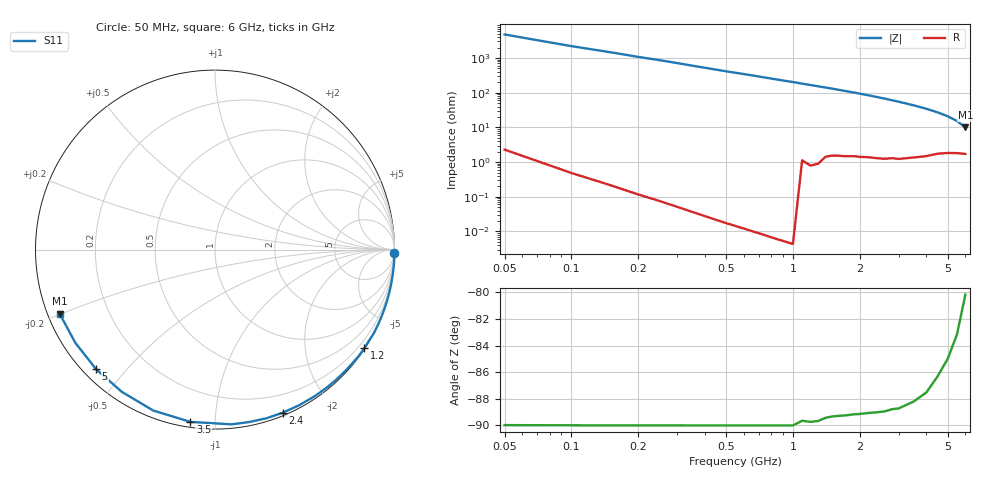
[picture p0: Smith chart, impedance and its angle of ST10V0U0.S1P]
! SIEMENS Discrete & RF Semiconductors
! BA892
! Si PIN Diode in SCD-80
! VR = 10 V
! S-Parameters:  September  1997
# GHz  S  MA  R  50
!  f  S11
! GHz  MAG  ANG
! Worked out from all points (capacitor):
!   34 points, 50 MHz to 6 GHz, reference 50 ohm
!   read as one part to ground: C = 722 fF near 50 MHz
!   lowest |Z| = 10 ohm at 6 GHz (marker M1)
!   S11 on the Smith chart (normalised r, x): 50 MHz: 0, -95; 1.2 GHz: 0.02, -3.33; 2.4 GHz: 0.03, -1.50; 3.5 GHz: 0.03, -0.87; 5 GHz: 0.04, -0.42; 6 GHz: 0.03, -0.20
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0.05  1 -1.2
0.25  1 -6.6
0.4  1 -10.9
0.5  1 -13.8
0.6  1 -16.5
0.7  1 -19.3
0.8  1 -22.2
0.9  1 -25.0
1  1 -27.7
1.2  0.9974 -33.4
1.3  0.9965 -36.2
1.5  0.9922 -41.7
1.6  0.9912 -44.6
1.7  0.9904 -47.5
1.8  0.9894 -50.3
1.9  0.9883 -53.1
2  0.9876 -56.0
2.2  0.9857 -61.7
2.4  0.9841 -67.5
2.6  0.9825 -73.2
2.8  0.9793 -78.9
3  0.978 -84.6
3.5  0.9696 -98.1
4  0.9604 -111.0
4.5  0.9474 -123.2
5  0.9396 -134.8
5.5  0.9356 -146.3
6  0.9362 -157.6
